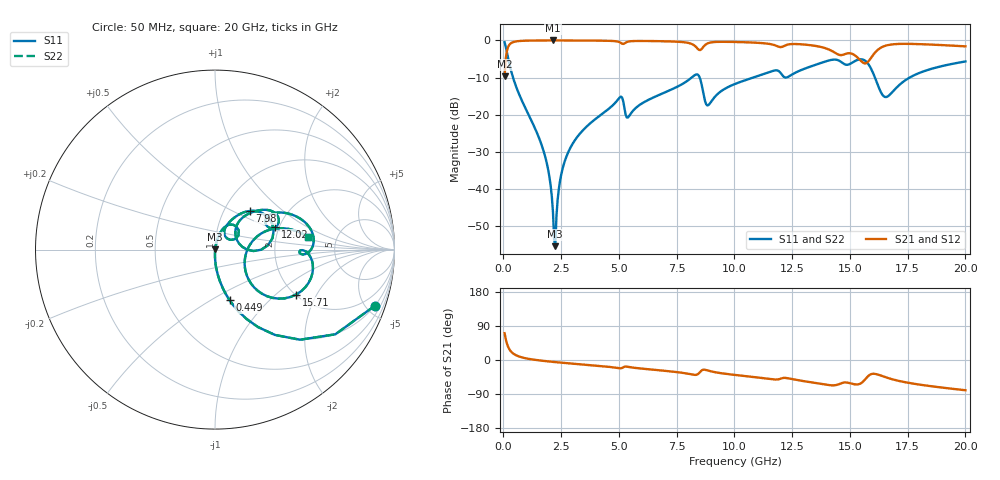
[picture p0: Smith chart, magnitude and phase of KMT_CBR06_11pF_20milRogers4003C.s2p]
! Data measured by Modelithics Inc. support@modelithics.com 813-866-6335
! KEMET CBR0603 11pF, Pad Width= 0.851mm, Pad Length= 0.64mm, Pad Gap= 0.62mm, 20mil Rogers 4003C substrate Data, January 2022
# hz S ma R 50
! 2 Port Network Data from SP1.SP block
! freq  magS11  angS11  magS21  angS21  magS12  angS12  magS22  angS22
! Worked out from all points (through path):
!   401 points, 50 MHz to 20 GHz, reference 50 ohm
!   highest |S21| = -0.01 dB at 2.145 GHz (marker M1); lowest = -9.7 dB at 50 MHz (marker M2)
!   group delay of S21, straight-line fit = 11.3 ps
!   lowest |S11| = -55.3 dB at 2.244 GHz (marker M3), VSWR 1.00, Z = 50.1 + j0.113 ohm
!   |S11| at or under -10 dB: 415.9 MHz to 8.144 GHz (7.728 GHz wide, 181 % of centre); 8.496 GHz to 10.81 GHz (2.313 GHz wide, 24 % of centre); 16.08 GHz to 17.58 GHz (1.499 GHz wide, 8.9 % of centre)
!   |S22| runs from -55.3 to -0.5 dB; largest |S21 - S12| = 0
!   S11 on the Smith chart (normalised r, x): 50 MHz: 0.99, -5.70; 449 MHz: 0.99, -0.61; 7.98 GHz: 1.31, +0.62; 12.02 GHz: 1.91, +0.55; 15.71 GHz: 2.02, -1.38; 20 GHz: 3.04, +0.60
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5e7  0.9442 -19.3  0.3292 70.6  0.3292 70.6  0.9442 -19.3
2.495e8  0.4937 -61.0  0.8691 29.0  0.8691 29.0  0.4937 -61.0
4.49e8  0.2931 -73.9  0.9554 15.9  0.9554 15.9  0.2931 -73.9
1.74575e9  0.03193 -90.5  0.9984 -2.4  0.9984 -2.4  0.03193 -90.5
1.995125e9  0.0143 -89.6  0.9987 -4.1  0.9987 -4.1  0.0143 -89.6
2.14475e9  0.004888 -81.3  0.9988 -5.0  0.9988 -5.0  0.004888 -81.3
2.2445e9  0.001713 40.9  0.9987 -5.6  0.9987 -5.6  0.001713 40.9
2.593625e9  0.02063 78.9  0.9984 -7.5  0.9984 -7.5  0.02063 78.9
3.391625e9  0.05964 76.8  0.9965 -11.7  0.9965 -11.7  0.05964 76.8
5.0375e9  0.1715 53.6  0.9429 -21.8  0.9429 -21.8  0.1715 53.6
5.386625e9  0.09201 49.6  0.9611 -18.0  0.9611 -18.0  0.09201 49.6
6.73325e9  0.1848 61.3  0.9772 -27.0  0.9772 -27.0  0.1848 61.3
7.980125e9  0.2889 48.1  0.9286 -36.1  0.9286 -36.1  0.2889 48.1
8.429e9  0.3441 18.2  0.762 -36.9  0.762 -36.9  0.3441 18.2
8.877875e9  0.1353 30.1  0.922 -28.2  0.922 -28.2  0.1353 30.1
1.0025e10  0.2597 47.9  0.953 -39.4  0.953 -39.4  0.2597 47.9
1.202e10  0.3594 20.4  0.814 -48.8  0.814 -48.8  0.3594 20.4
1.336662e10  0.4536 26.3  0.8568 -59.3  0.8568 -59.3  0.4536 26.3
1.571075e10  0.5173 -28.9  0.4954 -47.5  0.4954 -47.5  0.5173 -28.9
1.62095e10  0.2513 -41.7  0.7485 -38.4  0.7485 -38.4  0.2513 -41.7
1.670825e10  0.1839 2.2  0.873 -48.6  0.873 -48.6  0.1839 2.2
2e10  0.5212 7.9  0.8322 -79.8  0.8322 -79.8  0.5212 7.9
